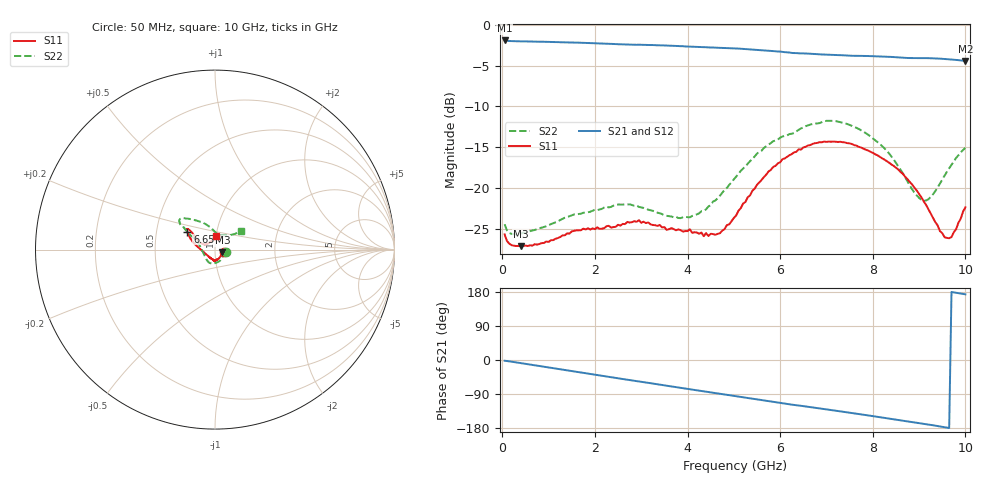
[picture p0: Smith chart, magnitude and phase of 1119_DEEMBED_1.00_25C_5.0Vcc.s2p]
!Hittite Microwave Corp.
!Digital Attenuator/PhaseShifter Rev 1.4.0
!Filename: C:\DATA\DATA\1119_DEEMBED_1.00_25C_5.0Vcc.s2p
!VNA ID: Agilent Technologies,N5224A,MY51441122,A.10.45.03
!Device type:
!2 Port Calibration.
!Temp(C): 25
!Lot Number:
!Serial Number:
!Operator:
!Misc:
!Attenuator:  1.000
# GHZ S DB R 50.0
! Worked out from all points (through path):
!   200 points, 50 MHz to 10 GHz, reference 50 ohm
!   highest |S21| = -1.94 dB at 50 MHz (marker M1); lowest = -4.4 dB at 10 GHz (marker M2)
!   group delay of S21, straight-line fit = 51 ps
!   lowest |S11| = -27.1 dB at 400 MHz (marker M3), VSWR 1.09, Z = 54.3 - j1.74 ohm
!   |S11| at or under -10 dB: start of sweep to end of sweep
!   |S22| runs from -25.6 to -11.7 dB; largest |S21 - S12| = 0.0019
!   S11 on the Smith chart (normalised r, x): 50 MHz: 1.11, -0.03; 6.65 GHz: 0.72, +0.15; 10 GHz: 1.00, +0.15
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0.05  -25.61 -16.8  -1.94 -1.9  -1.93 -1.9  -24.38 -14.3
0.15  -26.74 -14.4  -2.01 -3.5  -2.00 -3.5  -25.43 -13.9
0.4  -27.05 -21.1  -2.05 -8.2  -2.04 -8.2  -25.51 -21.9
1.75  -24.91 -75.6  -2.23 -34.1  -2.22 -34.1  -22.97 -76.2
2.65  -24.36 -87.8  -2.44 -51.1  -2.43 -51.1  -21.93 -108.5
2.95  -23.88 -93.3  -2.46 -56.5  -2.46 -56.5  -22.26 -120.1
3.4  -24.46 -100.6  -2.53 -65.0  -2.53 -65.0  -23.03 -135.4
3.85  -25.09 -106.5  -2.64 -73.5  -2.63 -73.5  -23.63 -151.8
4.25  -25.54 -116.7  -2.74 -80.8  -2.75 -80.9  -23.04 -172.6
4.7  -25.47 -145.7  -2.84 -89.2  -2.86 -89.2  -20.89 164.1
5.05  -23.30 -171.3  -2.92 -95.7  -2.93 -95.8  -18.56 153.9
5.85  -17.38 159.8  -3.24 -110.8  -3.25 -110.8  -14.24 146.4
6.65  -14.71 146.9  -3.56 -124.4  -3.56 -124.4  -12.21 143.2
6.7  -14.57 146.7  -3.58 -125.3  -3.58 -125.3  -12.14 142.7
7.45  -14.47 143.0  -3.78 -138.2  -3.78 -138.2  -12.14 134.9
8.35  -16.85 145.1  -3.94 -154.6  -3.94 -154.6  -15.72 113.7
8.9  -19.91 153.0  -4.09 -164.4  -4.08 -164.4  -20.53 87.7
9.15  -22.00 155.8  -4.10 -169.2  -4.10 -169.2  -21.48 69.6
9.45  -25.21 146.1  -4.16 -175.3  -4.17 -175.3  -19.42 47.9
9.65  -26.08 122.3  -4.25 -179.5  -4.25 -179.5  -17.55 39.6
9.799999  -24.98 102.7  -4.32 177.4  -4.32 177.4  -16.28 37.0
10  -22.30 87.3  -4.43 173.3  -4.43 173.3  -15.06 35.6
